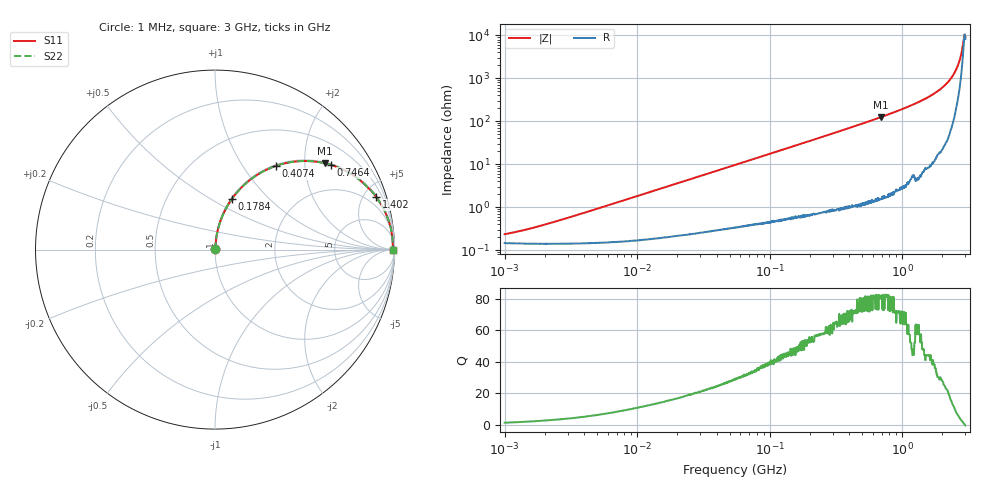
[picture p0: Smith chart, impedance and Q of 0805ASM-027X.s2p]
!s-Parameter Generated by FASTRON Sdn. Bhd.
!FASTRON P/N : 0805ASM-027X
!Keysight Technologies: E4991B_MY54100416_A.01.15
!Date: Fri Jun 19 14:48:09 2026
!Version  :Rev00  Fri Jun 19 14:48:09 2026
!Data & Calibration Information:
!Freq  S11  S21  S12  S22
!PortZ  Port1:50+j0  Port2:50+j0
!When reading reference impedance value at option line is always used.
! Remarks : This data is being provided solely for informational purposes.
# Hz S dB R 50
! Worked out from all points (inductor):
!   1601 points, 1 MHz to 3 GHz, reference 50 ohm
!   read as one part in series: L = 29.1 nH near 2.318 MHz
!   highest Q = 81.7 at 695.9 MHz (marker M1), where L = 28.8 nH
!   self-resonance near 2.955 GHz
!   S11 on the Smith chart (normalised r, x): 1 MHz: 1.00, +0.00; 178.4 MHz: 1.01, +0.62; 407.4 MHz: 1.02, +1.43; 746.4 MHz: 1.03, +2.72; 1.402 GHz: 1.12, +6.08; 3 GHz: open
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1000000  -52.60 51.3  -0.01 -0.1  -0.01 -0.1  -52.60 51.3
1691165  -49.40 65.4  -0.01 -0.2  -0.01 -0.2  -49.40 65.4
3804036  -43.00 77.9  -0.01 -0.4  -0.01 -0.4  -43.00 77.9
1.447069e7  -31.70 84.3  -0.02 -1.5  -0.02 -1.5  -31.70 84.3
5.504702e7  -20.40 82.5  -0.07 -5.5  -0.07 -5.5  -20.40 82.5
1.013595e8  -15.20 78.6  -0.17 -10.0  -0.17 -10.0  -15.20 78.6
1.784169e8  -10.60 71.7  -0.45 -17.1  -0.45 -17.1  -10.60 71.7
2.083556e8  -9.42 69.2  -0.59 -19.8  -0.59 -19.8  -9.42 69.2
2.913464e8  -6.95 62.4  -1.05 -26.7  -1.05 -26.7  -6.95 62.4
4.073935e8  -4.78 54.0  -1.84 -35.2  -1.84 -35.2  -4.78 54.0
6.958997e8  -2.18 38.2  -4.17 -51.1  -4.17 -51.1  -2.18 38.2
7.463997e8  -1.93 36.1  -4.60 -53.2  -4.60 -53.2  -1.93 36.1
7.925923e8  -1.73 34.2  -4.99 -55.0  -4.99 -55.0  -1.73 34.2
1.402151e9  -0.49 18.1  -10.20 -70.8  -10.20 -70.8  -0.49 18.1
1.893158e9  -0.21 10.7  -14.70 -77.4  -14.70 -77.4  -0.21 10.7
2.124078e9  -0.14 7.9  -17.20 -79.6  -17.20 -79.6  -0.14 7.9
2.347656e9  -0.10 5.5  -20.30 -80.7  -20.30 -80.7  -0.10 5.5
2.51802e9  -0.08 3.9  -23.40 -79.9  -23.40 -79.9  -0.08 3.9
2.660507e9  -0.08 2.6  -26.80 -76.9  -26.80 -76.9  -0.08 2.6
2.75535e9  -0.08 1.8  -29.90 -72.0  -29.90 -72.0  -0.08 1.8
2.896736e9  -0.08 0.6  -37.10 -47.3  -37.10 -47.3  -0.08 0.6
3e9  -0.08 -0.3  -39.40 26.0  -39.40 26.0  -0.08 -0.3
